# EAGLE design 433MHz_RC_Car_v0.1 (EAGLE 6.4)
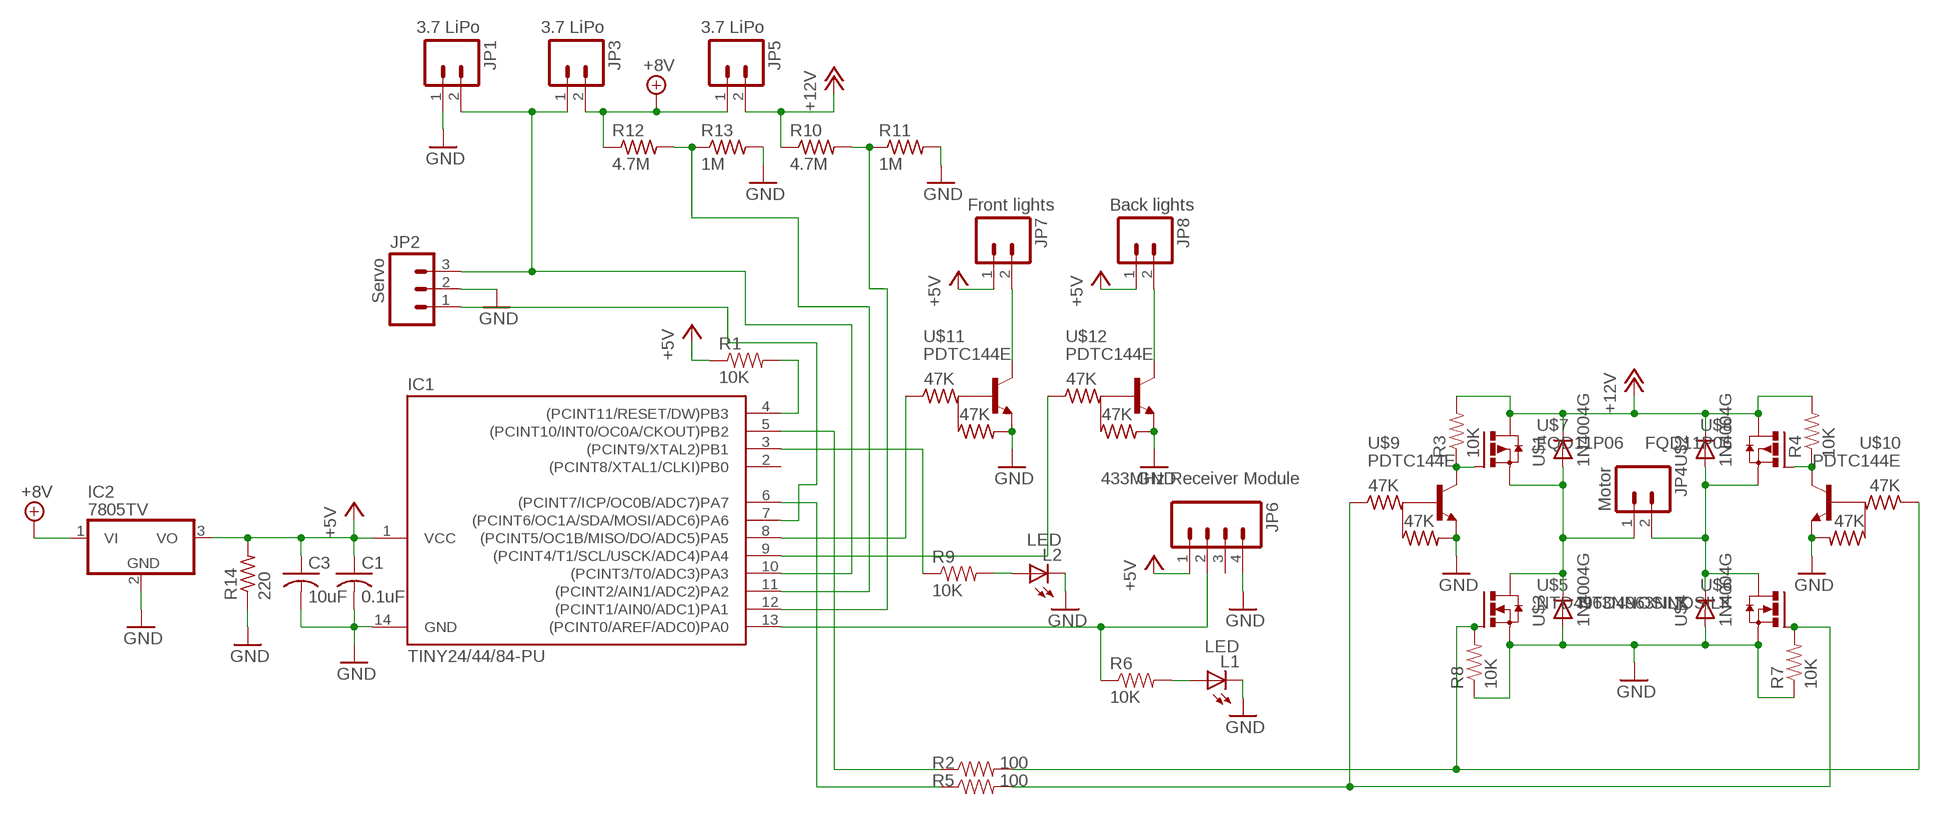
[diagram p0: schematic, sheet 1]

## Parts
C1  0.1uF  C-US025-024X044  [C025-024X044]
C3  10uF  C-US  [C050-50D]
IC1  TINY24/44/84-PU  [DIL14]
IC2  7805TV  [TO220V]
JP1  3.7 LiPo  M02PTH  [1X02]
JP2  Servo  M03PTH  [1X03]
JP3  3.7 LiPo  M02PTH  [1X02]
JP4  Motor  M02PTH  [1X02]
JP5  3.7 LiPo  M02PTH  [1X02]
JP6  433MHz Receiver Module  M04433MHZ  [433MHZ_1X04]
JP7  Front lights  M02PTH  [1X02]
JP8  Back lights  M02PTH  [1X02]
L1  LED  LED3MM  [LED3MM]
L2  LED  LED3MM  [LED3MM]
R1  10K  RESISTOR5MM  [RESISTOR5MM]
R2  100  RESISTOR5MM  [RESISTOR5MM]
R3  10K  RESISTOR5MM  [RESISTOR5MM]
R4  10K  RESISTOR5MM  [RESISTOR5MM]
R5  100  RESISTOR5MM  [RESISTOR5MM]
R6  10K  RESISTOR5MM  [RESISTOR5MM]
R7  10K  RESISTOR5MM  [RESISTOR5MM]
R8  10K  RESISTOR5MM  [RESISTOR5MM]
R9  10K  RESISTOR5MM  [RESISTOR5MM]
R10  4.7M  R-US_R0805_2  [R0805_2]
R11  1M  R-US_R0805_2  [R0805_2]
R12  4.7M  R-US_R0805_2  [R0805_2]
R13  1M  R-US_R0805_2  [R0805_2]
R14  220  R-US_R0805_2  [R0805_2]
U$1  1N4004G  [1N4004G]
U$2  1N4004G  [1N4004G]
U$3  1N4004G  [1N4004G]
U$4  1N4004G  [1N4004G]
U$5  NTD4963NNOSILK  [TO220-1]
U$6  NTD4963NNOSILK  [TO220-1]
U$7  FQD11P06  [TO220-1]
U$8  FQD11P06  [TO220-1]
U$9  PDTC144E  [SOT23]
U$10  PDTC144E  [SOT23]
U$11  PDTC144E  [SOT23]
U$12  PDTC144E  [SOT23]

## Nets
+5V: C1.1 C3.1 IC1.1(VCC) IC2.3(VO) JP6.1 JP7.1 JP8.1 R1.P$1 R14.2
+8V: IC2.1(VI) JP3.2 JP5.1 R12.1
+12V: JP5.2 R3.P$2 R4.P$2 R10.1 U$1.C U$2.C U$7.3(S) U$8.3(S)
GND: C1.2 C3.2 IC1.14(GND) IC2.2(GND) JP1.1 JP2.2 JP6.4 L1.K(C) L2.K(C) R7.P$1 R8.P$1 R11.2 R13.2 R14.1 U$3.A U$4.A U$5.3(S) U$6.3(S) U$9.2(E) U$10.2(E) U$11.2(E) U$12.2(E)
N$1: IC1.7((PCINT6/OC1A/SDA/MOSI/ADC6)PA6) JP2.1
N$2: IC1.5((PCINT10/INT0/OC0A/CKOUT)PB2) R2.P$1
N$3: R4.P$1 U$8.1(G) U$10.3(C)
N$4: R3.P$1 U$7.1(G) U$9.3(C)
N$5: IC1.6((PCINT7/ICP/OC0B/ADC7)PA7) R5.P$1
N$7: IC1.8((PCINT5/OC1B/MISO/DO/ADC5)PA5) U$11.1(B)
N$8: IC1.10((PCINT3/T0/ADC3)PA3) JP1.2 JP2.3 JP3.1
N$9: IC1.9((PCINT4/T1/SCL/USCK/ADC4)PA4) U$12.1(B)
N$10: L1.A R6.P$2
N$11: IC1.3((PCINT9/XTAL2)PB1) R9.P$1
N$12: L2.A R9.P$2
N$13: JP7.2 U$11.3(C)
N$14: JP8.2 U$12.3(C)
N$15: IC1.12((PCINT1/AIN0/ADC1)PA1) R10.2 R11.1
N$16: IC1.11((PCINT2/AIN1/ADC2)PA2) R12.2 R13.1
N$20: JP4.2 U$2.A U$4.C U$6.2(D) U$8.2(D)
N$23: JP4.1 U$1.A U$3.C U$5.2(D) U$7.2(D)
N$26: R2.P$2 R8.P$2 U$5.1(G) U$10.1(B)
N$30: R5.P$2 R7.P$2 U$6.1(G) U$9.1(B)
RESET: IC1.4((PCINT11/RESET/DW)PB3) R1.P$2
RF_OUTPUT: IC1.13((PCINT0/AREF/ADC0)PA0) JP6.2 R6.P$1
Unconnected: IC1.2((PCINT8/XTAL1/CLKI)PB0) JP6.3

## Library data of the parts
C1 C3 = adafruit:C-US: CAPACITOR, American symbol
IC1 = avr-5:TINY24/44/84
IC2 = linear:78*: Positive VOLTAGE REGULATOR Source: http://cache.national.com/ds/LM/LM78L05.pdf http://www.fairchildsemi.com/ds/LM/LM7805.pdf
JP1 JP3-JP5 JP7 JP8 = SparkFun:M02: Header 2
JP2 = SparkFun:M03: Header 3 Standard 3-pin 0.1" header. Use with straight break away headers (SKU : PRT-00116), right angle break away headers (PRT-00553), swiss pins (PRT-00743), machine pins (PRT-00117), and female headers (PRT-00115). Molex polarized connector foot print use with SKU : PRT-08232 with associated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
JP6 = SparkFun:M04: Header 4 Standard 4-pin 0.1" header. Use with straight break away headers (SKU : PRT-00116), right angle break away headers (PRT-00553), swiss pins (PRT-00743), machine pins (PRT-00117), and female headers (PRT-00115). Molex polarized connector foot print use with SKU : PRT-08231 with associated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
L1 L2 = SparkFun:LED: LEDs
R1-R9 = SparkFun:RESISTOR: Resistor
R10-R14 = adafruit:R-US_: RESISTOR, American symbol
U$1-U$4 = alex:1N4004G
U$5 U$6 = transistor-fet_old:NTD4963N
U$7 U$8 = transistor-fet_old:FQD11P06
U$9-U$12 = transistor-npn:PDTC144E

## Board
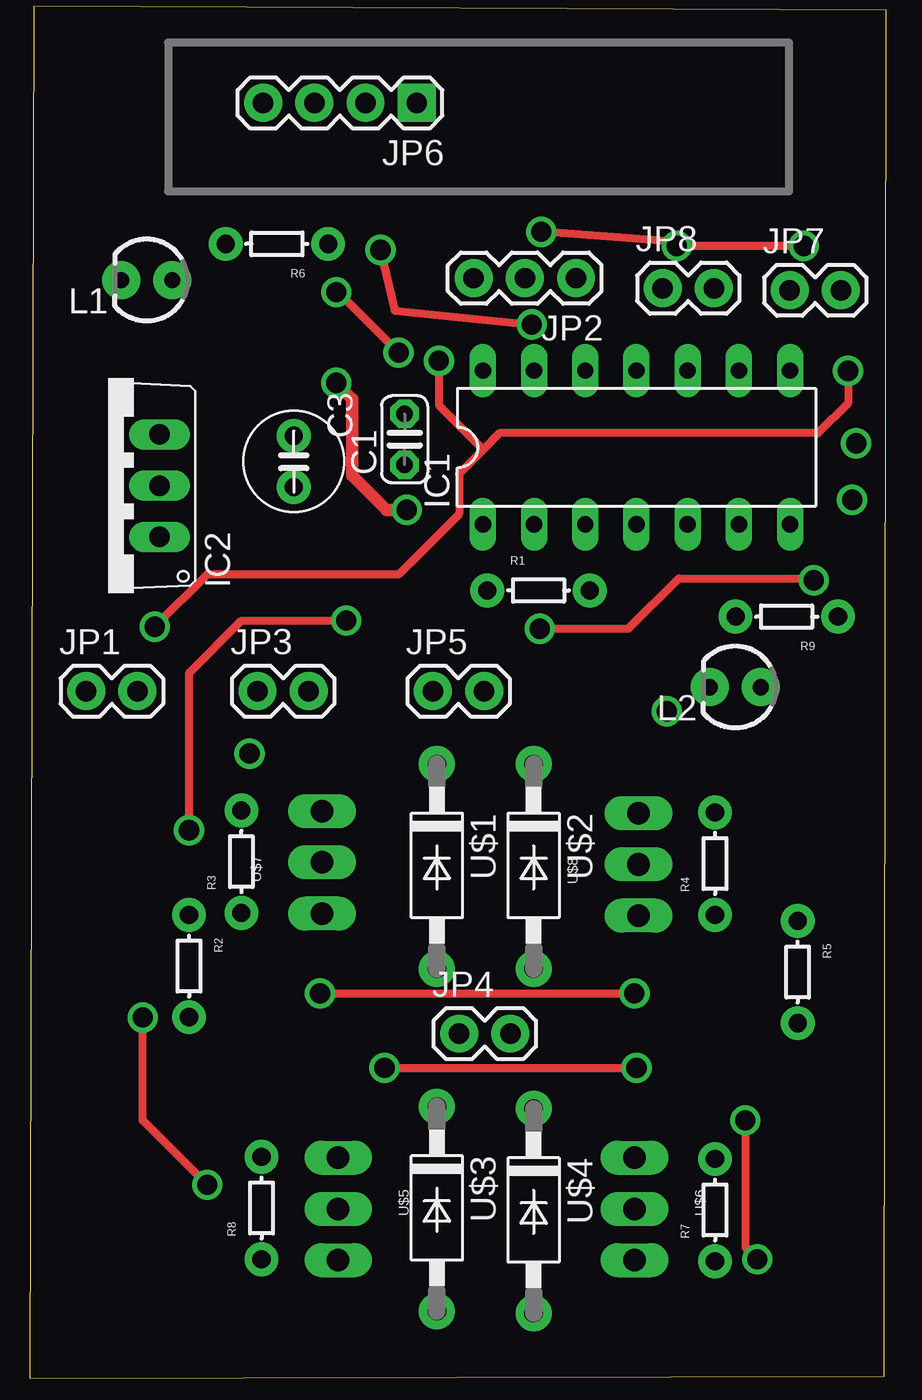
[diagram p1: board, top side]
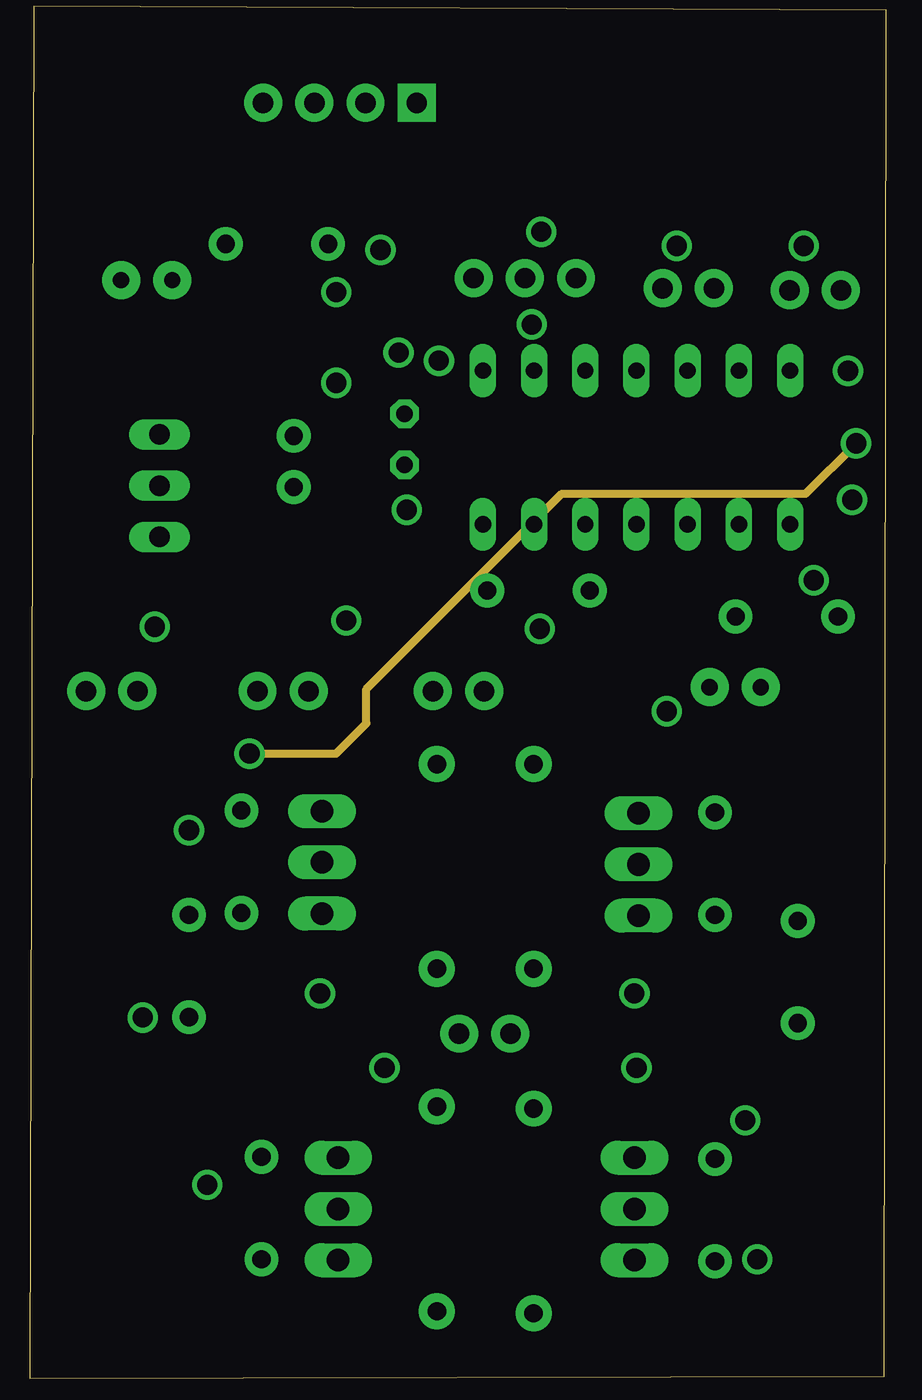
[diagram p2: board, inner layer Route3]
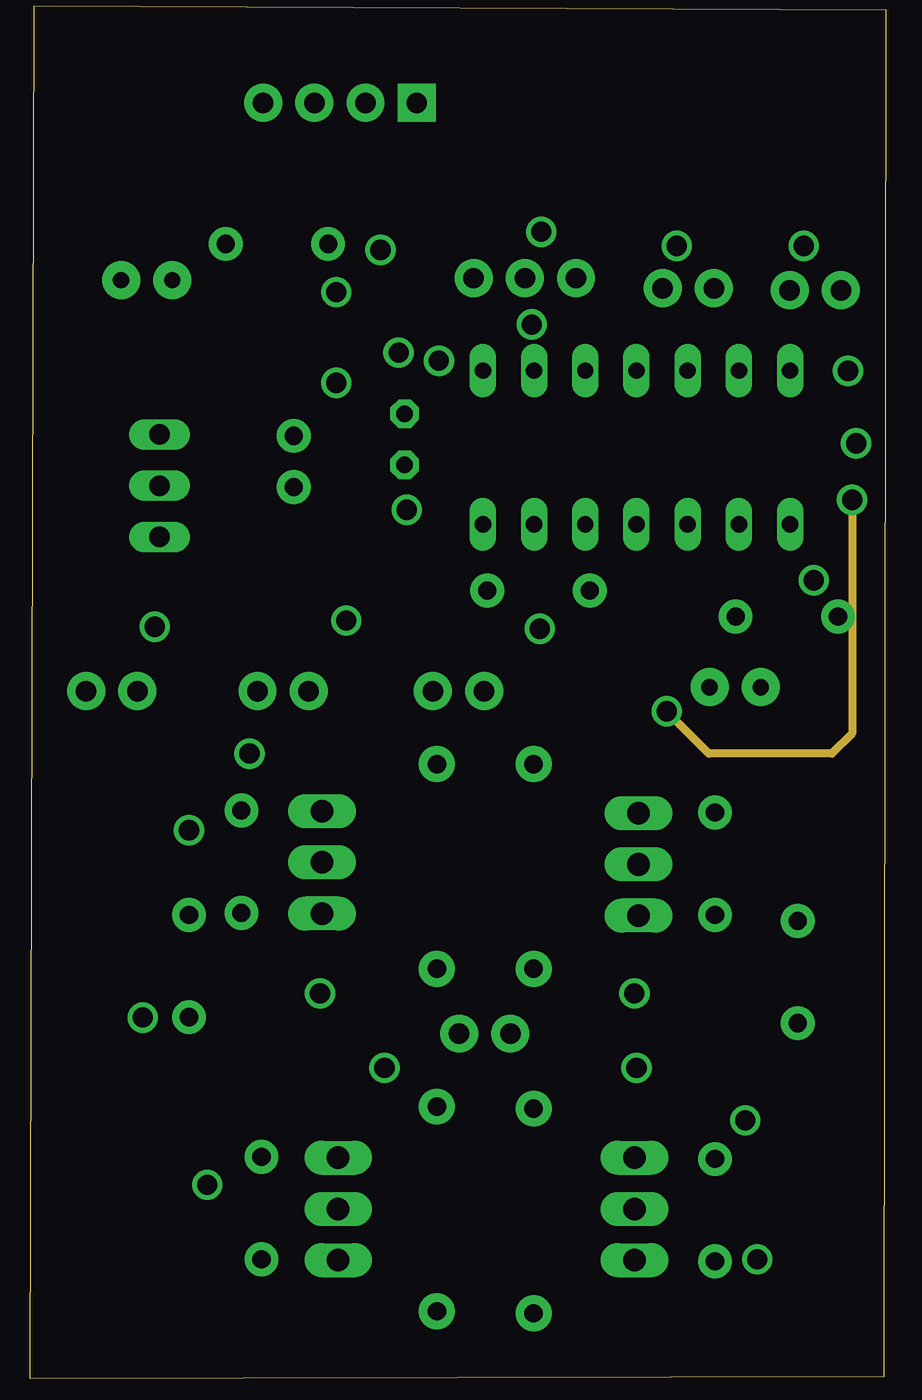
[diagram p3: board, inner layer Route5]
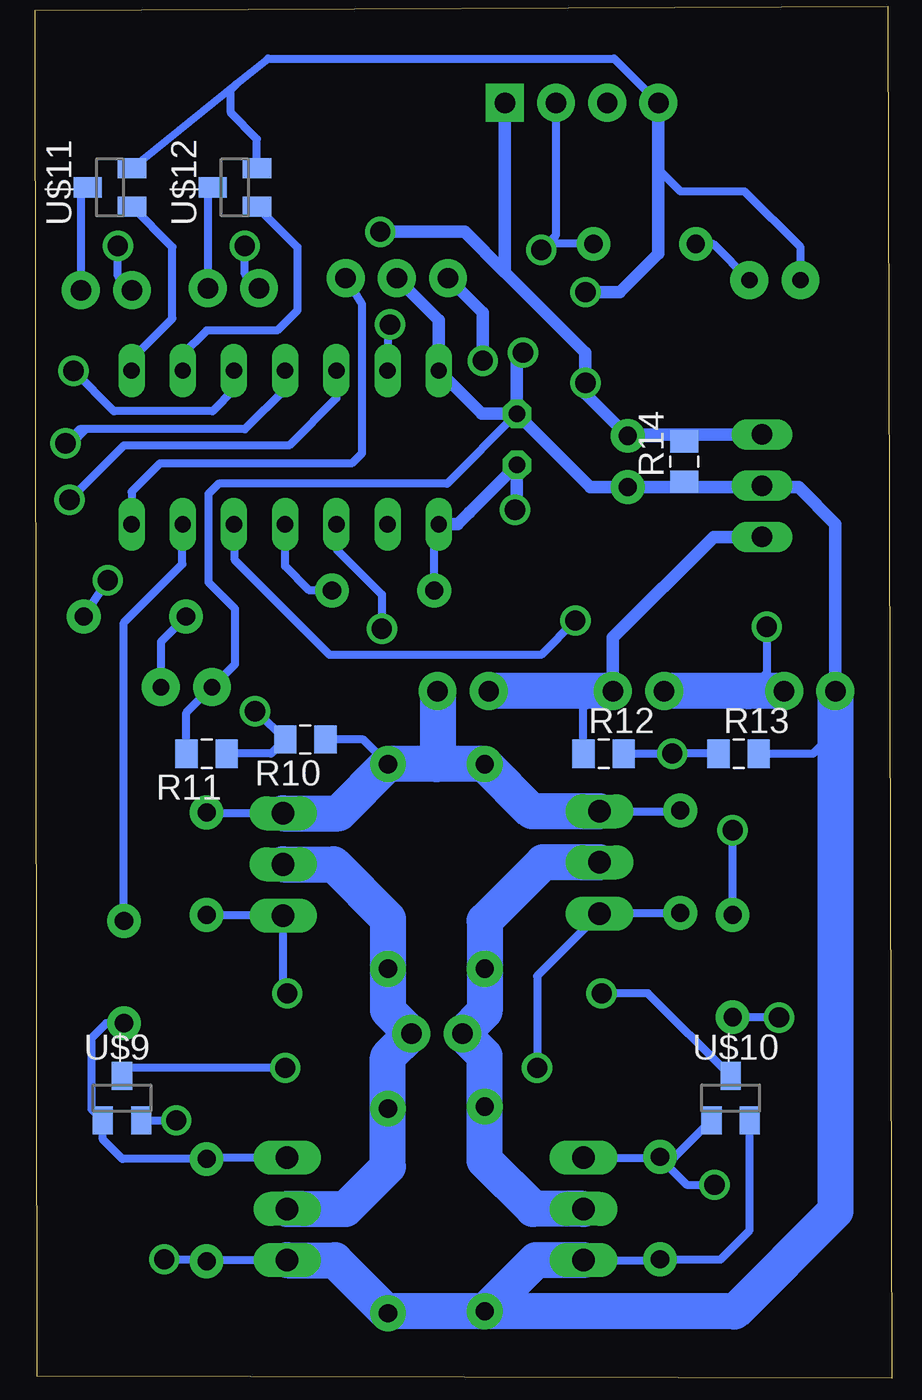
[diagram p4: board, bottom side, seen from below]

No outline drawn. Coordinates in mm, seen from the top.
Copper layers (1*16): Top 0.035mm / dielectric 1.5mm / Bottom 0.035mm
Design rules "Fusion_eagle_rule_v1.1": minimum track width 6mil, minimum drill 12mil, track to track 6mil, track to pad 6mil, pad to pad 6mil, via to via 6mil, smd to smd 0mil, copper to edge 10mil, drill to drill 10mil, minimum pad ring 10mil, minimum via ring 6mil, stop-mask expansion 2mil, vias tented up to drill 100mil, thermal gap 10mil
Milling: 4 lines

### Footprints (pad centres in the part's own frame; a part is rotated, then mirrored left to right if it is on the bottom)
C025-024X044 = drill 0.813 pad 1.422 octagon: 1 -1.27,0; 2 1.27,0
C050-50D = drill 0.9 pad 1.676: 1 -1.27,0; 2 1.27,0
DIL14 = drill 0.813 long: 1 -7.62,-3.81; 2 -5.08,-3.81; 3 -2.54,-3.81; 4 0,-3.81; 5 2.54,-3.81; 6 5.08,-3.81; 7 7.62,-3.81; 8 7.62,3.81; 9 5.08,3.81; 10 2.54,3.81; 11 0,3.81; 12 -2.54,3.81; 13 -5.08,3.81; 14 -7.62,3.81
TO220V = drill 1.016 long: 1 -2.54,-2.54; 2 0,-2.54; 3 2.54,-2.54
1X02 = drill 1.016 pad 1.88: 1 0,0; 2 2.54,0
1X03 = drill 1.016 pad 1.88: 1 0,0; 2 2.54,0; 3 5.08,0
433MHZ_1X04 = drill 1.016 pad 1.88 square: 1 0,0 | drill 1.016 pad 1.88: 2 2.54,0; 3 5.08,0; 4 7.62,0
LED3MM = drill 0.813 pad 1.88: A -1.27,0; K 1.27,0
RESISTOR5MM = drill 0.9 pad 1.676: P$1 -2.5,0; P$2 2.58,0
R0805_2 = smd 1.1 x 1.4: 1 -1,0; 2 1,0
1N4004G = drill 0.91 pad 1.778: A 5.08,0; C -5.08,0
TO220-1 = drill 1.118 long: 1 -2.54,0; 2 0,0; 3 2.54,0
SOT23 = smd 1 x 1.4: 1 -0.95,-1.1; 2 0.95,-1.1; 3 0,1.1

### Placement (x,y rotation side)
C1  25.8,32.2 90 top
C3  20.3,31.1 270 top
IC1  37.3,31.8 0 top
IC2  11.1,29.9 90 top
JP1  10,19.7 0 top
JP2  34.3,40.2 180 top
JP3  18.5,19.7 0 top
JP4  28.5,2.7 0 top
JP5  27.2,19.7 0 top
JP6  26.4,48.9 180 top
JP7  44.9,39.6 0 top
JP8  38.6,39.7 0 top
L1  13,40.1 180 top
L2  42.2,19.9 180 top
R1  32.4,24.7 0 top
R2  15.1,6.1 270 top
R3  17.7,11.2 90 top
R4  41.2,11.1 90 top
R5  45.3,5.8 270 top
R6  19.5,41.9 180 top
R7  41.2,-6.1 90 top
R8  18.7,-6 90 top
R9  44.8,23.4 180 top
R10  36.3,17.3 180 bottom
R11  41.2,16.6 180 bottom
R12  21.5,16.6 0 bottom
R13  14.8,16.6 0 bottom
R14  17.5,31.1 90 bottom
U$1  27.4,11 270 top
U$2  32.2,11 270 top
U$3  27.4,-6 270 top
U$4  32.2,-6.1 270 top
U$5  22.5,-6 270 top
U$6  37.2,-6 270 top
U$7  21.7,11.2 90 top
U$8  37.4,11.1 90 top
U$9  45.4,-0.5 0 bottom
U$10  15.2,-0.5 0 bottom
U$11  46,44.7 90 bottom
U$12  39.8,44.7 90 bottom

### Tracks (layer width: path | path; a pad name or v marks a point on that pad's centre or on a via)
+5V  (via drill 1)
  Top 0.406: v32.58,42.5 39.1,42 v39.3,41.8 v45.6,41.8
  Top 0.61: v25.9,28.7 24.9,28.7 23.2,30.4 23.2,34.2 v22.4,35
  Bottom 0.406: 28.5,28.23 28.16,28.57 | JP8.1 39.3,40.4 v39.3,41.8 | JP7.1 45.6,40.3 v45.6,41.8 | R1.P$1 29.9,27.77 IC1.1 | R14.2 17.77,32.37 C3.1
  Bottom 0.61: IC1.1 28.74,27.99 28.16,28.57 C1.1 25.8,28.8 v25.9,28.7 | IC2.3 20.23,32.44 C3.1 22.4,34.47 v22.4,35 22.4,36.5 26.4,40.5 | v32.58,42.5 28.4,42.5 26.4,40.5 | JP6.1 26.4,40.5
+8V
  Bottom 0.406: R12.1 22.5,19.6 22.4,19.7
  Bottom 0.61: JP3.2 21.04,22.36 16.04,27.36 IC2.1
  Bottom 1.778: JP3.2 22.4,19.7 JP5.1
+12V
  Bottom 0.406: U$7.3 17.74,13.74 R3.P$2 | U$8.3 41.16,13.64 R4.P$2 | U$2.C 33.42,17.3 R10.1
  Bottom 1.778: U$7.3 25.06,13.74 U$1.C 29.8,16.08 | U$8.3 34.64,13.64 U$2.C 29.8,16.08 | JP5.2 29.74,16.14 29.8,16.08
GND  (via drill 1)
  Top 0.406: v42.7,-1.6 42.7,-7.9 v43.3,-8.5 | v22.4,39.5 22.7,39.3 v25.5,36.5
  Bottom 0.406: U$6.3 41.14,-8.54 R7.P$1 41.3,-8.5 v43.3,-8.5 | U$5.3 18.74,-8.54 R8.P$1 15.7,-8.5 14.25,-7.05 U$10.2 | U$9.2 v42.7,-1.6 | JP6.4 20.98,51.1 38.15,51.1 39.71,49.84 | L1.K 11.73,41.73 14.5,44.5 17.68,44.5 18.78,45.6 | C1.2 29.27,30 40.6,30 41.1,29.5 41.1,25.1 39.8,23.8 39.8,21.03 L2.K 42.2,18.63 R11.2 | U$11.2 39.71,49.84 | U$12.2 38.7,47.1 40,48.4 40,49.55 39.71,49.84 | R13.2 11.1,16.6 10,17.7 | R14.1 17.77,29.83 19.7,29.83
  Bottom 0.61: C1.2 22.16,29.83 C3.2 19.7,29.83 13.71,29.83 | 29.8,35.73 IC1.14 | JP6.4 18.78,45.6 18.78,41.42 20.7,39.5 v22.4,39.5 | IC2.2 13.71,29.83 | JP1.1 10,28 11.83,29.83 13.71,29.83 | 25.4,36.6 v25.5,36.5 25.8,36.2 C1.2 | JP2.2 29.68,38.12 IC1.14 | IC1.14 27.54,33.47 C1.2
  Bottom 1.778: U$5.3 24.86,-8.54 U$3.A | U$6.3 34.84,-8.54 U$4.A 32.1,-11.08 U$3.A | JP1.1 10,17.7 10,-6.1 15,-11.1 15.02,-11.08 U$3.A
N$1
  Bottom 0.406: IC1.7 44.92,29.6 43.52,31 34,31 33.5,31.5 33.5,38.9 JP2.1
N$2  (via drill 1)
  Top 0.406: v15.1,12.8 15.1,20.6 17.7,23.2 v22.9,23.2
  Bottom 0.406: R2.P$1 v15.1,12.8 | IC1.5 39.8,27.95 39.8,26.2 35.1,21.5 24.6,21.5 v22.9,23.2
N$3  (via drill 1)
  Top 0.406: v21.6,4.7 v37.2,4.7
  Bottom 0.406: R4.P$1 41.16,8.56 U$8.1 37.4,4.9 v37.2,4.7 | U$10.3 19.3,4.7 v21.6,4.7
N$4  (via drill 1)
  Top 0.406: v24.8,1 v37.3,1
  Bottom 0.406: R3.P$1 21.66,8.7 U$7.1 24.8,5.56 v24.8,1 | v37.3,1 45,1 U$9.3
N$5
  Bottom 0.406: R5.P$1 45.3,23.1 42.4,26 42.4,27.97 IC1.6
N$7
  Bottom 0.406: 44.9,35.63 IC1.8 44.92,36.18 42.9,38.2 42.9,41.75 U$11.1
N$8  (via drill 1)
  Top 0.406: v47.8,35.6 47.8,34 46.3,32.5 30.5,32.5 29.7,31.7 | 29.7,31.7 28.5,30.5 28.5,28.5 25.5,25.5 16,25.5 v13.4,22.9 | v27.5,36.1 27.5,33.9 29.7,31.7
  Bottom 0.406: IC1.10 39.84,34.66 40.9,33.6 45.8,33.6 v47.8,35.6 | v13.4,22.9 13.4,20.6 14.3,19.7
  Bottom 0.61: JP2.3 27.5,38.48 v27.5,36.1
  Bottom 1.778: JP1.2 14.3,19.7 JP3.1
N$9
  Bottom 0.406: IC1.9 42.38,36.42 41.2,37.6 37.7,37.6 36.7,38.6 36.7,41.75 U$12.1
N$10
  Bottom 0.406: R6.P$2 16.07,41.9 L1.A
N$11  (via drill 1)
  Top 0.406: v32.5,22.8 36.9,22.8 39.4,25.3 46,25.3 v46.1,25.2
  Bottom 0.406: IC1.3 34.76,26.76 32.5,24.5 v32.5,22.8 | v46.1,25.2 47.4,23.3 R9.P$1
N$12
  Bottom 0.406: R9.P$2 43.47,22.15 L2.A
N$13
  Bottom 0.406: U$11.3 47.44,44.36 JP7.2
N$14
  Bottom 0.406: U$12.3 41.14,44.46 JP8.2
N$15  (via drill 1)
  Route5 0.406: v48,29.2 48,17.6 47,16.6 40.9,16.6 v38.8,18.7
  Bottom 0.406: R11.1 38,16.6 R10.2 38.7,18.7 v38.8,18.7 | IC1.12 34.76,34.24 37.1,31.9 45.3,31.9 v48,29.2
N$16  (via drill 1)
  Route3 0.406: v18.1,16.6 22.4,16.6 23.9,18.1 23.9,19.8 33.6,29.5 45.7,29.5 v48.2,32
  Bottom 0.406: IC1.11 37.3,34.7 39.3,32.7 47.2,32.7 | 47.2,32.7 47.5,32.7 v48.2,32 47.9,32 47.2,32.7 | R13.1 v18.1,16.6 R12.2
N$20
  Bottom 1.778: U$8.2 34.9,11.1 32.2,8.4 U$2.A 32.2,3.86 JP4.2 32.2,1.54 U$4.C 32.2,-3.9 34.3,-6 U$6.2
N$23
  Bottom 1.778: U$7.2 24.5,11.2 27.4,8.3 U$1.A 27.4,3.8 JP4.1 27.4,1.6 U$3.C 27.4,-3.6 25,-6 U$5.2
N$26  (via drill 1)
  Top 0.406: v16,-4.8 12.8,-1.6 v12.8,3.5
  Bottom 0.406: U$5.1 18.74,-3.46 R8.P$2 | R8.P$2 18.7,-3.48 17.38,-4.8 v16,-4.8 | U$10.1 17.97,-3.42 R8.P$2 | v12.8,3.5 12.82,3.52 R2.P$2
N$30
  Bottom 0.406: U$6.1 41.14,-3.46 R7.P$2 45.38,-3.52 46.35,-2.55 U$9.1 46.9,-1.05 46.9,2.5 46.18,3.22 R5.P$2
RESET
  Bottom 0.406: IC1.4 37.3,25.9 36.1,24.7 R1.P$2
RF_OUTPUT  (via drill 1)
  Top 0.406: v24.6,41.6 25.3,38.6 v32.1,37.9
  Bottom 0.406: JP6.2 23.86,42.34 v24.6,41.6 24.3,41.9 R6.P$1 | v32.1,37.9 32.22,37.78 IC1.13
